(* Logix 5000 AddOnInstructionDefinition export Banner_S15C_B21_Param_v4; software revision 33.00 *)

TYPE Banner_Black_Host_Out_Mirroring :
STRUCT
   Enable : SINT;   // 0=Disabled, 1=Enabled
   Port_Selection : SINT;   // 0=Port 1
   Channel_Selection : SINT;   // 0=Discrete 1, 1=Discrete 2
   Inversion : SINT;   // 0=Not Inverted, 1=Inverted
   Polarity : SINT;   // 0=NPN Output, 1=PNP Output
   Output_Type : SINT;   // 1=Output Open Collector, 2=Output Push Pull
END_STRUCT
END_TYPE

TYPE Banner_Direct_v4 :
STRUCT
   Master_Cycle_Time : INT;
   Min_Cycle_Time : INT;
   M_Sequence_Capability : INT;
   IO_Link_Version_ID : INT;
   Process_Data_Input_Length : INT;
   Process_Data_Output_Length : INT;
   Combined_Vendor_ID : DINT;   // IO-Link Vendor ID
   Vendor_ID1 : INT;
   Vendor_ID2 : INT;
   Combined_Device_ID : DINT;   // IO-Link Device ID
   Device_ID1 : INT;
   Device_ID2 : INT;
   Device_ID3 : INT;
END_STRUCT
END_TYPE

TYPE Banner_Discrete_Host_Out_Mirroring_Cfg :
STRUCT
   Enable : SINT;   // 0=Disabled, 1=Enabled.
   Port_Selection : SINT;   // 0=Port 1
   Channel_Selection : SINT;   // 0=Discrete 1, 1=Discrete 2.
   Mirroring_Inversion : SINT;   // 0=Not Inverted, 1=Inverted.
   Mirroring_Polarity : SINT;   // 0=NPN Output, 1=PNP Output.
   Output_Type : SINT;   // 0=Output with Internal Pull Up / Down, 1=Output Open Collector, 2=Output Push Pull.
END_STRUCT
END_TYPE

TYPE Banner_IO_Metrics_v4 :
STRUCT
   Port_1_DI1_Count : DINT;
   Port_1_DI1_Duration : DINT;
   Port_1_DI1_Events_per_Minute : DINT;
   Port_1_DI1_Counts_per_Minute : DINT;
   Port_1_DI1_Totalizer_Counter : DINT;
   Port_1_DI2_Count : DINT;
   Port_1_DI2_Duration : DINT;
   Port_1_DI2_Events_per_Minute : DINT;
   Port_1_DI2_Counts_per_Minute : DINT;
   Port_1_DI2_Totalizer_Counter : DINT;
END_STRUCT
END_TYPE

TYPE Banner_IOL_Port_v4 :   // UDT that has all of the data items necessary to communicate with a specific Port on a IO-Link Master
STRUCT
   Port_Controlled : INT;   // Each bit represents a port on an IO-Link Master. Set to 1 to tell AOI to control that port.
   Port_Activate : INT;   // Each bit represents a port on an IO-Link Master. When ON that port will process any commands in queue.
   Port_Read : INT;   // Each bit represents a port on an IO-Link Master. Used to determine when device AOI has requested a Read command.
   Port_Write : INT;   // Each bit represents a port on an IO-Link Master. Used to determine when device AOI has requested a Write command.
   Port_RW_Complete : INT;   // Each bit represents a port on an IO-Link Master. Tells device AOI that Read or Write request has been completed.
   Port_Device_Read : INT;
   Data_Transfer : SINT[190];   // Array to transfer data from IO-Master to device AOIs.
END_STRUCT
END_TYPE

TYPE Banner_S15C_B21_Port_Config_v4 :
STRUCT
   DI1_IO_Selection : SINT;   // 0=NPN, 1=PNP
   DI1_Delay_Mode : SINT;   // 0=Disabled, 1=On Off Delay, 2=On One-Shot, 3=Off One-Shot, 4=On Pulse Stretcher, 5=Off Pulse Stretcher, 6=Totalizer
   DI1_Delay_Timer_1 : DINT;   // On Delay, One-Shot, Pulse Stretcher or Totalizer count.
   DI1_Delay_Timer_2 : DINT;   // Off Delay or Totalizer count.
   DI2_IO_Selection : SINT;   // 0=NPN, 1=PNP
   DI2_Delay_Mode : SINT;   // 0=Disabled, 1=On Off Delay, 2=On One-Shot, 3=Off One-Shot, 4=On Pulse Stretcher, 5=Off Pulse Stretcher, 6=Totalizer
   DI2_Delay_Timer_1 : DINT;   // On Delay, One-Shot, Pulse Stretcher or Totalizer count.
   DI2_Delay_Timer_2 : DINT;   // Off Delay or Totalizer count.
   Mirroring_Enable : SINT;   // 0=Disabled, 1=Enabled
   Mirroring_Port_Selection : SINT;   // 0 = Port 1
   Mirroring_Channel_Selection : SINT;   // 0=Discrete 1, 1=Discrete 2.
   Mirroring_Inversion : SINT;   // 0=Not Inverted, 1=Inverted
   Counts_per_Minute_Mode : SINT;   // 0=Slow, 1=Medium, 2=Fast
END_STRUCT
END_TYPE

TYPE Banner_S15C_B21_RD_v4 :   // All of the read parameters for a S15C unit.
STRUCT
   Direct : Banner_Direct_v4;
   Serial_Number : STRING;
   Product_Name : STRING;
   All_Time_Run_Time : DINT;   // Current All Time Run Timer.
   IO_Metrics : Banner_IO_Metrics_v4;
END_STRUCT
END_TYPE

TYPE Banner_S15C_B21_v4 :   // All of the parameters for a S15C.
STRUCT
   Initial_Global_Read : BOOL;   // Determines if all of the IO-Link data has been read into the PLC yet
   Command : INT;   // Value placed in here will activate a read or write to a specifc IO-Link Index
   Read : Banner_S15C_B21_RD_v4;   // Read Only Data
   Write : Banner_S15C_B21_WD_v4;   // Write Data
   Archive : Banner_S15C_B21_WD_v4;   // Archive Data
   Reset : BOOL;   // Resets AOI. This will force a complete parameter read of the sensor.
END_STRUCT
END_TYPE

TYPE Banner_S15C_B21_VSC_v4 :   // Vendor Specific Configuration Parameter Data for S15C-B21 unit.
STRUCT
   PDI1_Metric_Selection : SINT;   // 0 = Disabled, 1 = Count, 2 = Duration, 3 = Events per Minute
   PDI1_Port_Selection : SINT;   // 0 = Port 1
   PDI1_Channel_Selection : SINT;   // 0 = Discrete 1, 1 = Discrete 2
   PDI2_Metric_Selection : SINT;   // 0 = Disabled, 1 = Count, 2 = Duration, 3 = Events per Minute
   PDI2_Port_Selection : SINT;   // 0 = Port 1
   PDI2_Channel_Selection : SINT;   // 0 = Discrete 1, 1 = Discrete 2
   PDI3_Metric_Selection : SINT;   // 0 = Disabled, 1 = Count, 2 = Duration, 3 = Events per Minute
   PDI3_Port_Selection : SINT;   // 0 = Port 1
   PDI3_Channel_Selection : SINT;   // 0 = Discrete 1, 1 = Discrete 2
   PDI4_Metric_Selection : SINT;   // 0 = Disabled, 1 = Count, 2 = Duration, 3 = Events per Minute
   PDI4_Port_Selection : SINT;   // 0 = Port 1
   PDI4_Channel_Selection : SINT;   // 0 = Discrete 1, 1 = Discrete 2
END_STRUCT
END_TYPE

TYPE Banner_S15C_B21_WD_v4 :   // UDT that stores the Write Data for a S15C unit.
STRUCT
   System_Command : INT;   // See IODD file for list of commands that can be activated via the System Command interface
   Parameter_Access_Lock : SINT;   // Write access to all parameters is prohibited while value is 1. Only this parameter can be adjusted when value is 1.
   Data_Storage_Lock : SINT;   // Automatic data storage is disabled when this value is equal to 1. Read access is not affected.
   Local_Parameterization_Lock : SINT;   // Parameterization via local control elements on device is disabled.
   Local_User_Interface_Lock : SINT;   // Operation of local user interface is disabled.
   Resetable_Run_Time : DINT;   // Current Resetable Run Timer.
   VSC : Banner_S15C_B21_VSC_v4;
   All_Time_Run_Time_Event_Time : DINT;   // Time before an Event is generated. 0 = disable all-time event.
   Resetable_Run_Time_Event_Time : DINT;   // Time before an Event is generated. 0 = disable run time event.
   Port_1_Discrete_1 : SINT;   // 1 = Reset Activate
   Port_1_Discrete_2 : SINT;   // 1 = Reset Activate
   Port_1_Discrete_1_Reset_Count : DINT;
   Port_1_Discrete_2_Reset_Count : DINT;
   Port_1_Configuration : Banner_S15C_B21_Port_Config_v4;
   Mirroring_Config : Banner_Discrete_Host_Out_Mirroring_Cfg;
   Black_Mirroring_Config : Banner_Black_Host_Out_Mirroring;
END_STRUCT
END_TYPE

ADD_ON_INSTRUCTION Banner_S15C_B21_Param_v4   (* revision 4.3, vendor Banner Engineering *)
// AOI to read and write parameter data to an IO-Link S15C-B21.
VAR_IN_OUT
   S15C : Banner_S15C_B21_v4; {required}
   Port_Data : Banner_IOL_Port_v4; {required}
END_VAR
VAR_INPUT
   Port : DINT; {required}
END_VAR
VAR
   Local_Control : DINT; {access None}
   Global_Read_Command_Value : INT; {access None}
   Global_Write_Command_Value : INT; {access None}
   Error_Generated : BOOL; {access None}
   Command_Being_Processed : BOOL; {access None}
   Index_Write_Inprocess : INT; {access None}
   Index_Write_Control : INT; {access None}
   Update_Archive : BOOL; {access None}
   Inprocess_Index : DINT; {access None}
END_VAR

ROUTINE Logic   (* ladder *)
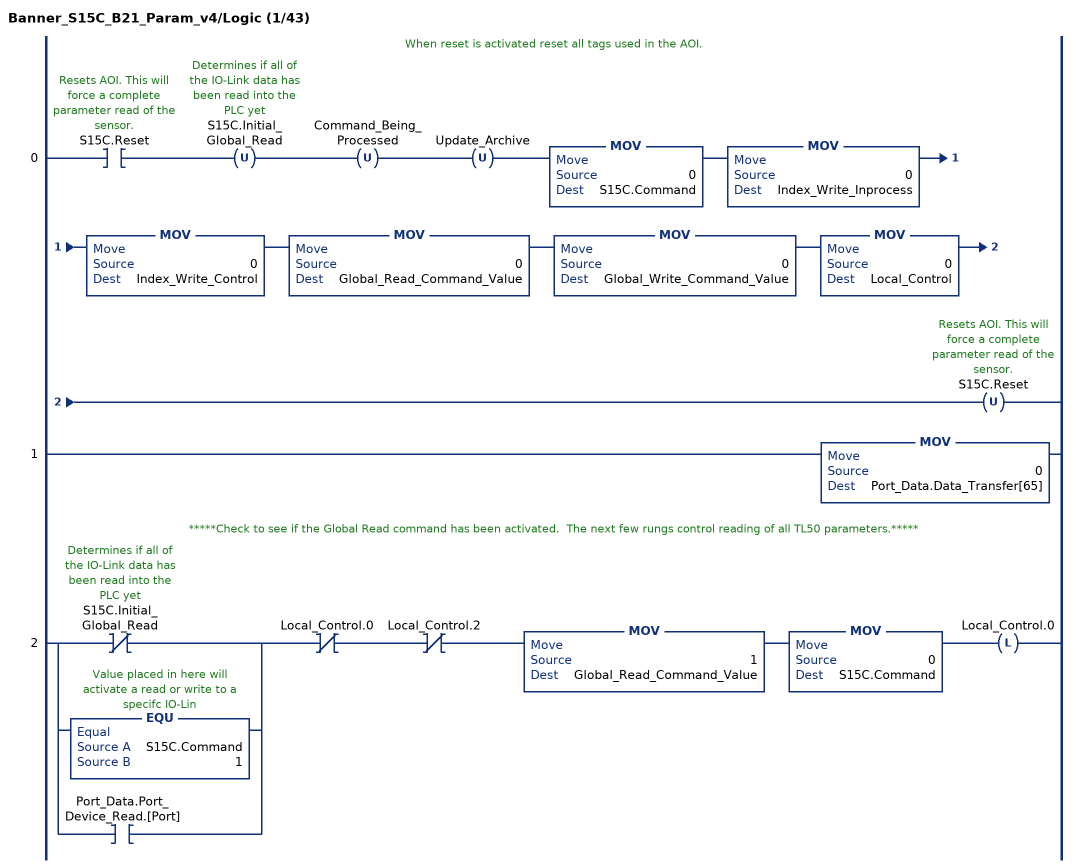
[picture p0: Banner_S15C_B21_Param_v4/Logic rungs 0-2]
   // When reset is activated reset all tags used in the AOI.
   0: XIC(S15C.Reset)OTU(S15C.Initial_Global_Read)OTU(Command_Being_Processed)OTU(Update_Archive)MOV(0,S15C.Command)MOV(0,Index_Write_Inprocess)MOV(0,Index_Write_Control)MOV(0,Global_Read_Command_Value)MOV(0,Global_Write_Command_Value)MOV(0,Local_Control)OTU(S15C.Reset);
   1: MOV(0,Port_Data.Data_Transfer[65]);
   // *****Check to see if the Global Read command has been activated.  The next few rungs control reading of all TL50 parameters.*****
   2: [XIO(S15C.Initial_Global_Read) ,EQU(S15C.Command,1) ,XIC(Port_Data.Port_Device_Read.[Port]) ]XIO(Local_Control.0)XIO(Local_Control.2)MOV(1,Global_Read_Command_Value)MOV(0,S15C.Command)OTL(Local_Control.0);
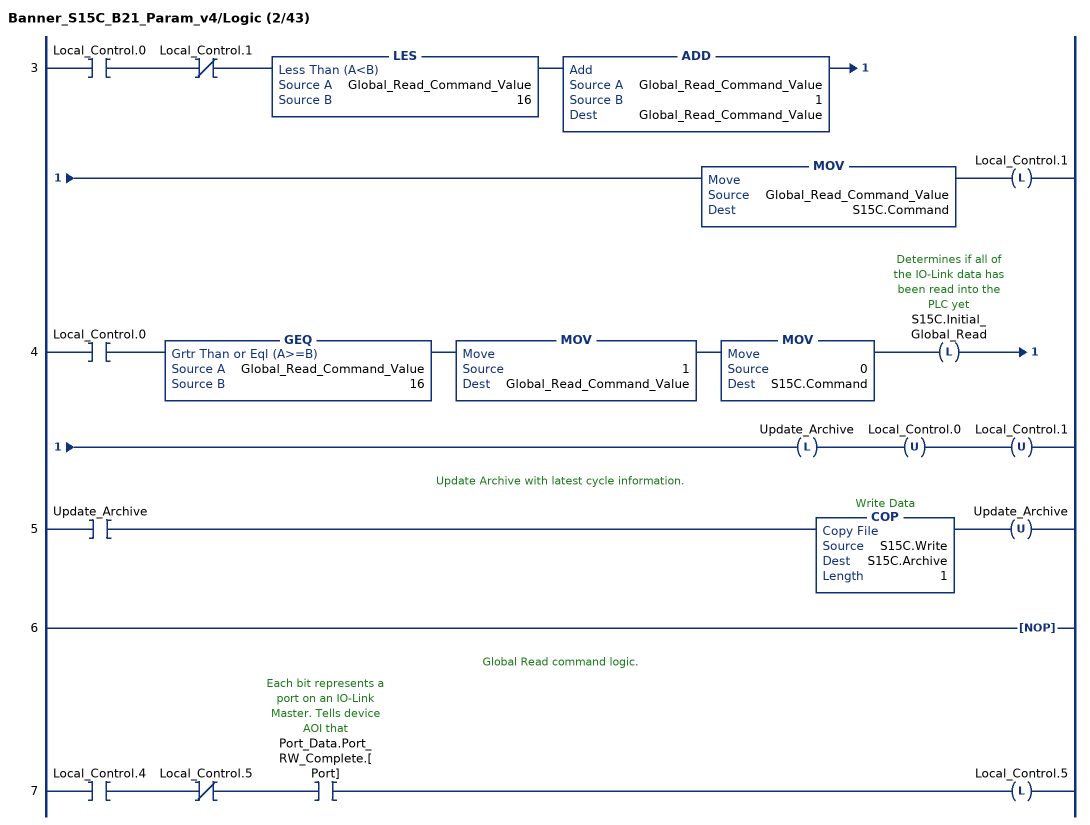
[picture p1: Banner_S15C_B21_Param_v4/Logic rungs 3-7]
   3: XIC(Local_Control.0)XIO(Local_Control.1)LES(Global_Read_Command_Value,16)ADD(Global_Read_Command_Value,1,Global_Read_Command_Value)MOV(Global_Read_Command_Value,S15C.Command)OTL(Local_Control.1);
   4: XIC(Local_Control.0)GEQ(Global_Read_Command_Value,16)MOV(1,Global_Read_Command_Value)MOV(0,S15C.Command)OTL(S15C.Initial_Global_Read)OTL(Update_Archive)OTU(Local_Control.0)OTU(Local_Control.1);
   // Update Archive with latest cycle information.
   5: XIC(Update_Archive)COP(S15C.Write,S15C.Archive,1)OTU(Update_Archive);
   6: NOP();
   // Global Read command logic.
   7: XIC(Local_Control.4)XIO(Local_Control.5)XIC(Port_Data.Port_RW_Complete.[Port])OTL(Local_Control.5);
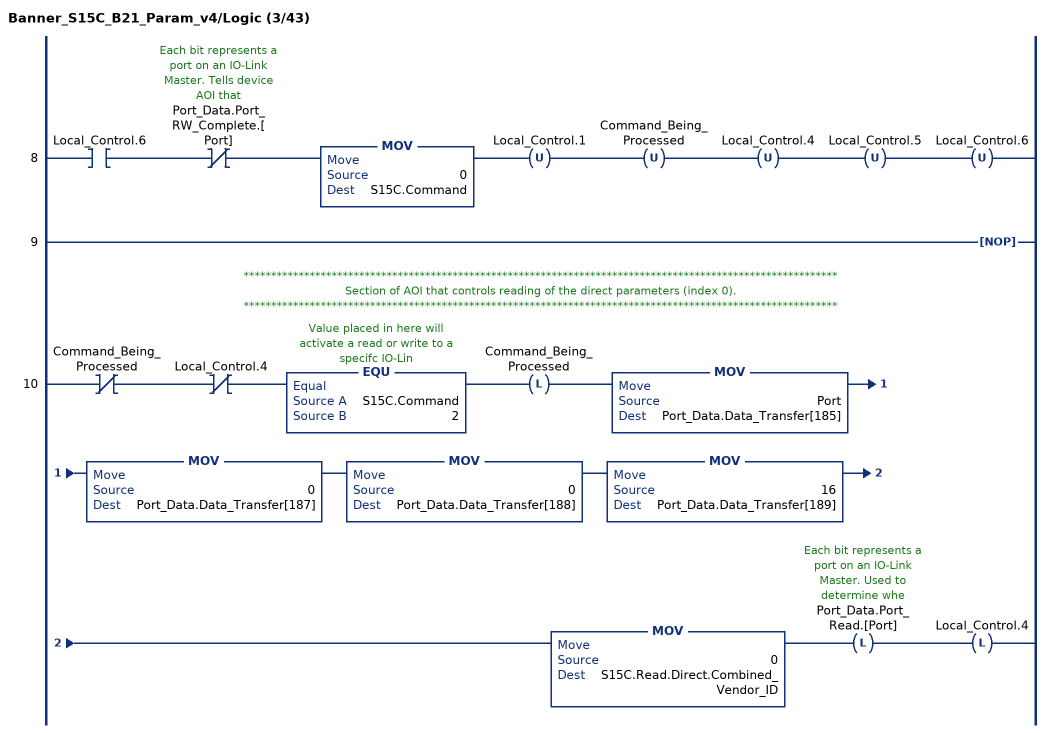
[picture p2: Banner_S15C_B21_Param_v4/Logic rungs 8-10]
   8: XIC(Local_Control.6)XIO(Port_Data.Port_RW_Complete.[Port])MOV(0,S15C.Command)OTU(Local_Control.1)OTU(Command_Being_Processed)OTU(Local_Control.4)OTU(Local_Control.5)OTU(Local_Control.6);
   9: NOP();
   // ************************************************************************************************************
   // Section of AOI that controls reading of the direct parameters (index 0).
   // ************************************************************************************************************
   10: XIO(Command_Being_Processed)XIO(Local_Control.4)EQU(S15C.Command,2)OTL(Command_Being_Processed)MOV(Port,Port_Data.Data_Transfer[185])MOV(0,Port_Data.Data_Transfer[187])MOV(0,Port_Data.Data_Transfer[188])MOV(16,Port_Data.Data_Transfer[189])MOV(0,S15C.Read.Direct.Combined_Vendor_ID)OTL(Port_Data.Port_Read.[Port])OTL(Local_Control.4);
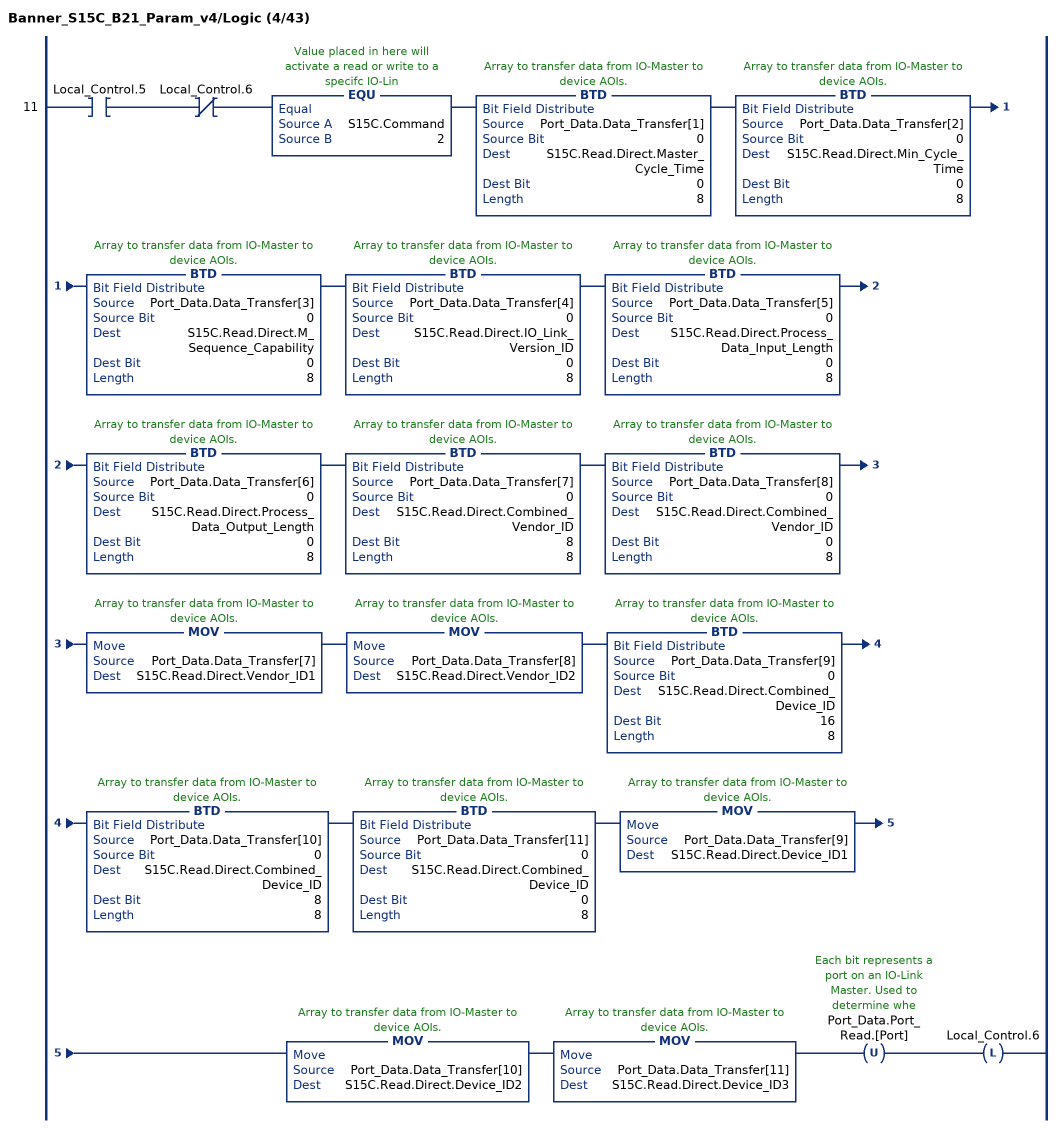
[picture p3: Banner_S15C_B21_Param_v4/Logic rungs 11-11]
   11: XIC(Local_Control.5)XIO(Local_Control.6)EQU(S15C.Command,2)BTD(Port_Data.Data_Transfer[1],0,S15C.Read.Direct.Master_Cycle_Time,0,8)BTD(Port_Data.Data_Transfer[2],0,S15C.Read.Direct.Min_Cycle_Time,0,8)BTD(Port_Data.Data_Transfer[3],0,S15C.Read.Direct.M_Sequence_Capability,0,8)BTD(Port_Data.Data_Transfer[4],0,S15C.Read.Direct.IO_Link_Version_ID,0,8)BTD(Port_Data.Data_Transfer[5],0,S15C.Read.Direct.Process_Data_Input_Length,0,8)BTD(Port_Data.Data_Transfer[6],0,S15C.Read.Direct.Process_Data_Output_Length,0,8)BTD(Port_Data.Data_Transfer[7],0,S15C.Read.Direct.Combined_Vendor_ID,8,8)BTD(Port_Data.Data_Transfer[8],0,S15C.Read.Direct.Combined_Vendor_ID,0,8)MOV(Port_Data.Data_Transfer[7],S15C.Read.Direct.Vendor_ID1)MOV(Port_Data.Data_Transfer[8],S15C.Read.Direct.Vendor_ID2)BTD(Port_Data.Data_Transfer[9],0,S15C.Read.Direct.Combined_Device_ID,16,8)BTD(Port_Data.Data_Transfer[10],0,S15C.Read.Direct.Combined_Device_ID,8,8)BTD(Port_Data.Data_Transfer[11],0,S15C.Read.Direct.Combined_Device_ID,0,8)MOV(Port_Data.Data_Transfer[9],S15C.Read.Direct.Device_ID1)MOV(Port_Data.Data_Transfer[10],S15C.Read.Direct.Device_ID2)MOV(Port_Data.Data_Transfer[11],S15C.Read.Direct.Device_ID3)OTU(Port_Data.Port_Read.[Port])OTL(Local_Control.6);
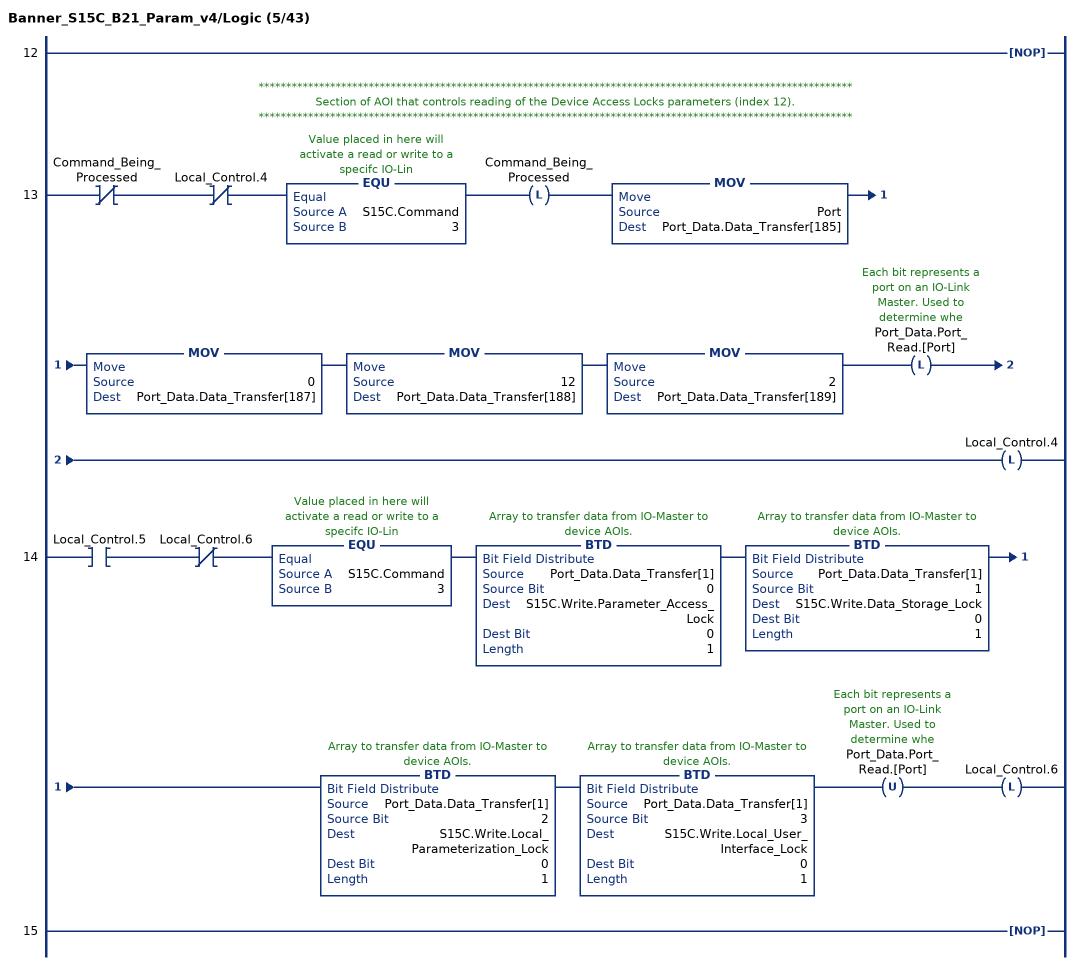
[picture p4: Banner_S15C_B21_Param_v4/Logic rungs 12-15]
   12: NOP();
   // ************************************************************************************************************
   // Section of AOI that controls reading of the Device Access Locks parameters (index 12).
   // ************************************************************************************************************
   13: XIO(Command_Being_Processed)XIO(Local_Control.4)EQU(S15C.Command,3)OTL(Command_Being_Processed)MOV(Port,Port_Data.Data_Transfer[185])MOV(0,Port_Data.Data_Transfer[187])MOV(12,Port_Data.Data_Transfer[188])MOV(2,Port_Data.Data_Transfer[189])OTL(Port_Data.Port_Read.[Port])OTL(Local_Control.4);
   14: XIC(Local_Control.5)XIO(Local_Control.6)EQU(S15C.Command,3)BTD(Port_Data.Data_Transfer[1],0,S15C.Write.Parameter_Access_Lock,0,1)BTD(Port_Data.Data_Transfer[1],1,S15C.Write.Data_Storage_Lock,0,1)BTD(Port_Data.Data_Transfer[1],2,S15C.Write.Local_Parameterization_Lock,0,1)BTD(Port_Data.Data_Transfer[1],3,S15C.Write.Local_User_Interface_Lock,0,1)OTU(Port_Data.Port_Read.[Port])OTL(Local_Control.6);
   15: NOP();
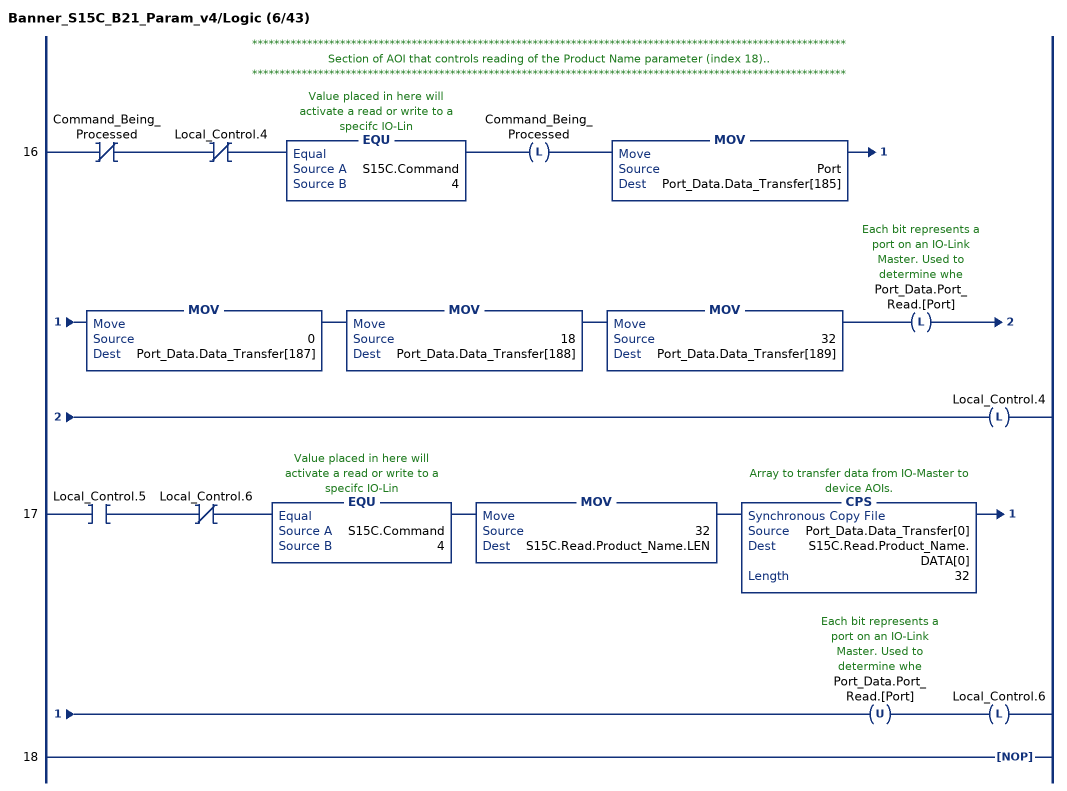
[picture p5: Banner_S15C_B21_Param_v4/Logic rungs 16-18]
   // ************************************************************************************************************
   // Section of AOI that controls reading of the Product Name parameter (index 18)..
   // ************************************************************************************************************
   16: XIO(Command_Being_Processed)XIO(Local_Control.4)EQU(S15C.Command,4)OTL(Command_Being_Processed)MOV(Port,Port_Data.Data_Transfer[185])MOV(0,Port_Data.Data_Transfer[187])MOV(18,Port_Data.Data_Transfer[188])MOV(32,Port_Data.Data_Transfer[189])OTL(Port_Data.Port_Read.[Port])OTL(Local_Control.4);
   17: XIC(Local_Control.5)XIO(Local_Control.6)EQU(S15C.Command,4)MOV(32,S15C.Read.Product_Name.LEN)CPS(Port_Data.Data_Transfer[0],S15C.Read.Product_Name.DATA[0],32)OTU(Port_Data.Port_Read.[Port])OTL(Local_Control.6);
   18: NOP();
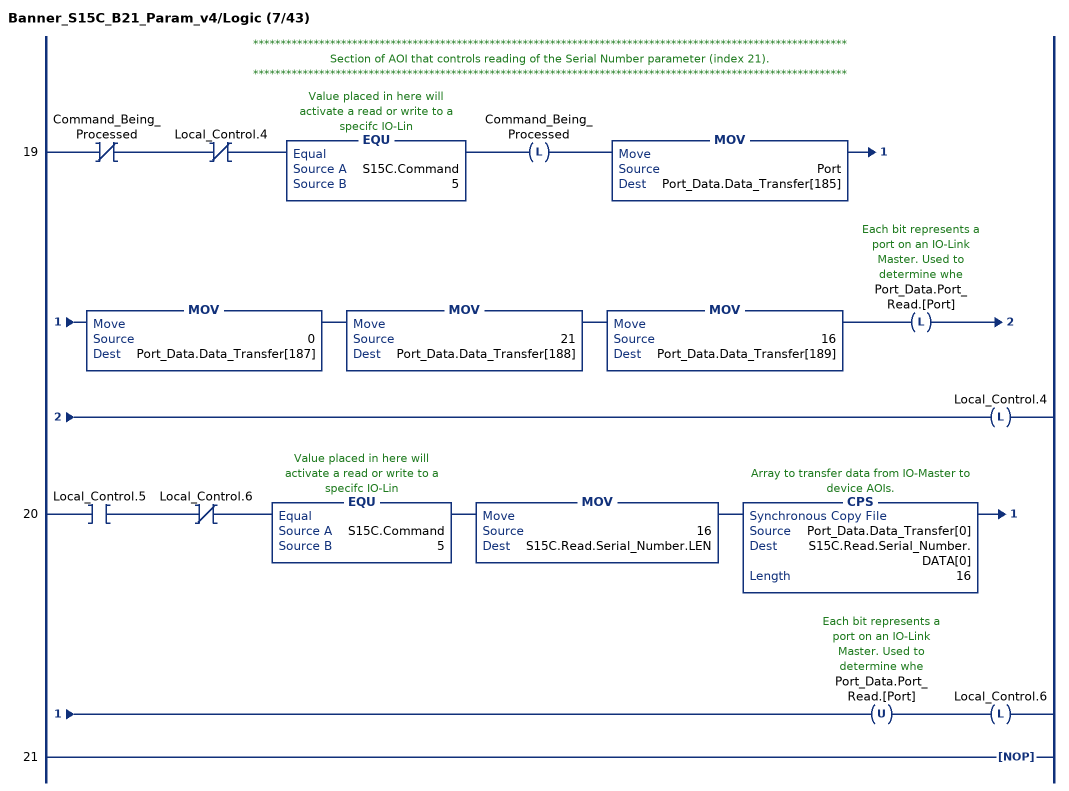
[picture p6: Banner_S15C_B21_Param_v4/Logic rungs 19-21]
   // ************************************************************************************************************
   // Section of AOI that controls reading of the Serial Number parameter (index 21).
   // ************************************************************************************************************
   19: XIO(Command_Being_Processed)XIO(Local_Control.4)EQU(S15C.Command,5)OTL(Command_Being_Processed)MOV(Port,Port_Data.Data_Transfer[185])MOV(0,Port_Data.Data_Transfer[187])MOV(21,Port_Data.Data_Transfer[188])MOV(16,Port_Data.Data_Transfer[189])OTL(Port_Data.Port_Read.[Port])OTL(Local_Control.4);
   20: XIC(Local_Control.5)XIO(Local_Control.6)EQU(S15C.Command,5)MOV(16,S15C.Read.Serial_Number.LEN)CPS(Port_Data.Data_Transfer[0],S15C.Read.Serial_Number.DATA[0],16)OTU(Port_Data.Port_Read.[Port])OTL(Local_Control.6);
   21: NOP();
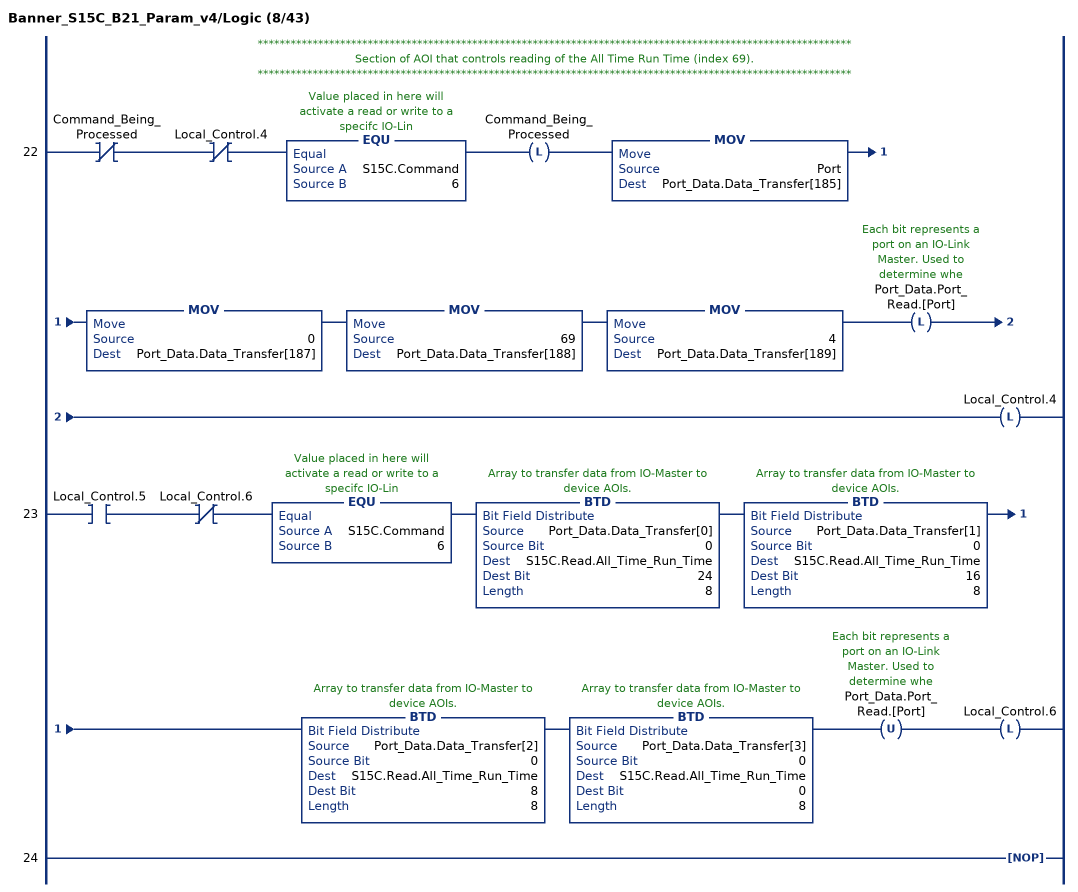
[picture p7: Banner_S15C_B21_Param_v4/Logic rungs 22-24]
   // ************************************************************************************************************
   // Section of AOI that controls reading of the All Time Run Time (index 69).
   // ************************************************************************************************************
   22: XIO(Command_Being_Processed)XIO(Local_Control.4)EQU(S15C.Command,6)OTL(Command_Being_Processed)MOV(Port,Port_Data.Data_Transfer[185])MOV(0,Port_Data.Data_Transfer[187])MOV(69,Port_Data.Data_Transfer[188])MOV(4,Port_Data.Data_Transfer[189])OTL(Port_Data.Port_Read.[Port])OTL(Local_Control.4);
   23: XIC(Local_Control.5)XIO(Local_Control.6)EQU(S15C.Command,6)BTD(Port_Data.Data_Transfer[0],0,S15C.Read.All_Time_Run_Time,24,8)BTD(Port_Data.Data_Transfer[1],0,S15C.Read.All_Time_Run_Time,16,8)BTD(Port_Data.Data_Transfer[2],0,S15C.Read.All_Time_Run_Time,8,8)BTD(Port_Data.Data_Transfer[3],0,S15C.Read.All_Time_Run_Time,0,8)OTU(Port_Data.Port_Read.[Port])OTL(Local_Control.6);
   24: NOP();
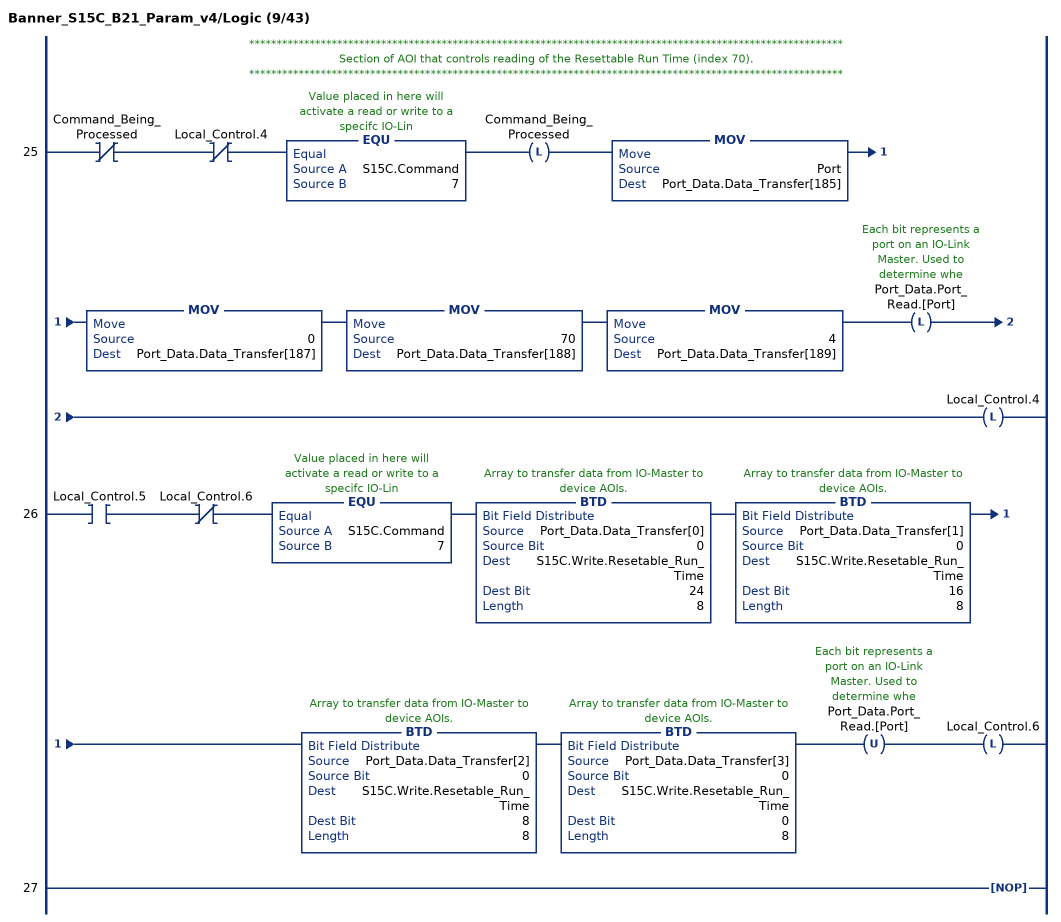
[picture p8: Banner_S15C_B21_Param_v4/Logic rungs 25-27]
   // ************************************************************************************************************
   // Section of AOI that controls reading of the Resettable Run Time (index 70).
   // ************************************************************************************************************
   25: XIO(Command_Being_Processed)XIO(Local_Control.4)EQU(S15C.Command,7)OTL(Command_Being_Processed)MOV(Port,Port_Data.Data_Transfer[185])MOV(0,Port_Data.Data_Transfer[187])MOV(70,Port_Data.Data_Transfer[188])MOV(4,Port_Data.Data_Transfer[189])OTL(Port_Data.Port_Read.[Port])OTL(Local_Control.4);
   26: XIC(Local_Control.5)XIO(Local_Control.6)EQU(S15C.Command,7)BTD(Port_Data.Data_Transfer[0],0,S15C.Write.Resetable_Run_Time,24,8)BTD(Port_Data.Data_Transfer[1],0,S15C.Write.Resetable_Run_Time,16,8)BTD(Port_Data.Data_Transfer[2],0,S15C.Write.Resetable_Run_Time,8,8)BTD(Port_Data.Data_Transfer[3],0,S15C.Write.Resetable_Run_Time,0,8)OTU(Port_Data.Port_Read.[Port])OTL(Local_Control.6);
   27: NOP();
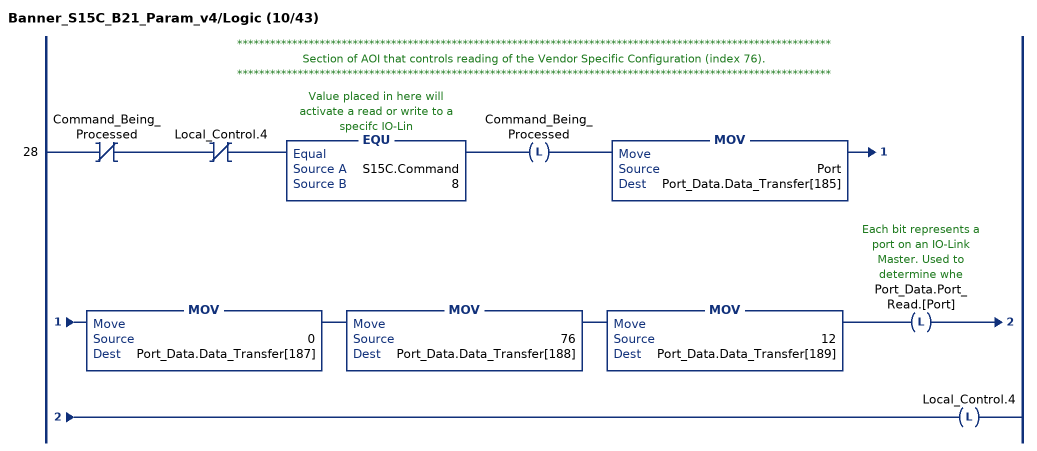
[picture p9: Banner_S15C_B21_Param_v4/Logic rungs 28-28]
   // ************************************************************************************************************
   // Section of AOI that controls reading of the Vendor Specific Configuration (index 76).
   // ************************************************************************************************************
   28: XIO(Command_Being_Processed)XIO(Local_Control.4)EQU(S15C.Command,8)OTL(Command_Being_Processed)MOV(Port,Port_Data.Data_Transfer[185])MOV(0,Port_Data.Data_Transfer[187])MOV(76,Port_Data.Data_Transfer[188])MOV(12,Port_Data.Data_Transfer[189])OTL(Port_Data.Port_Read.[Port])OTL(Local_Control.4);
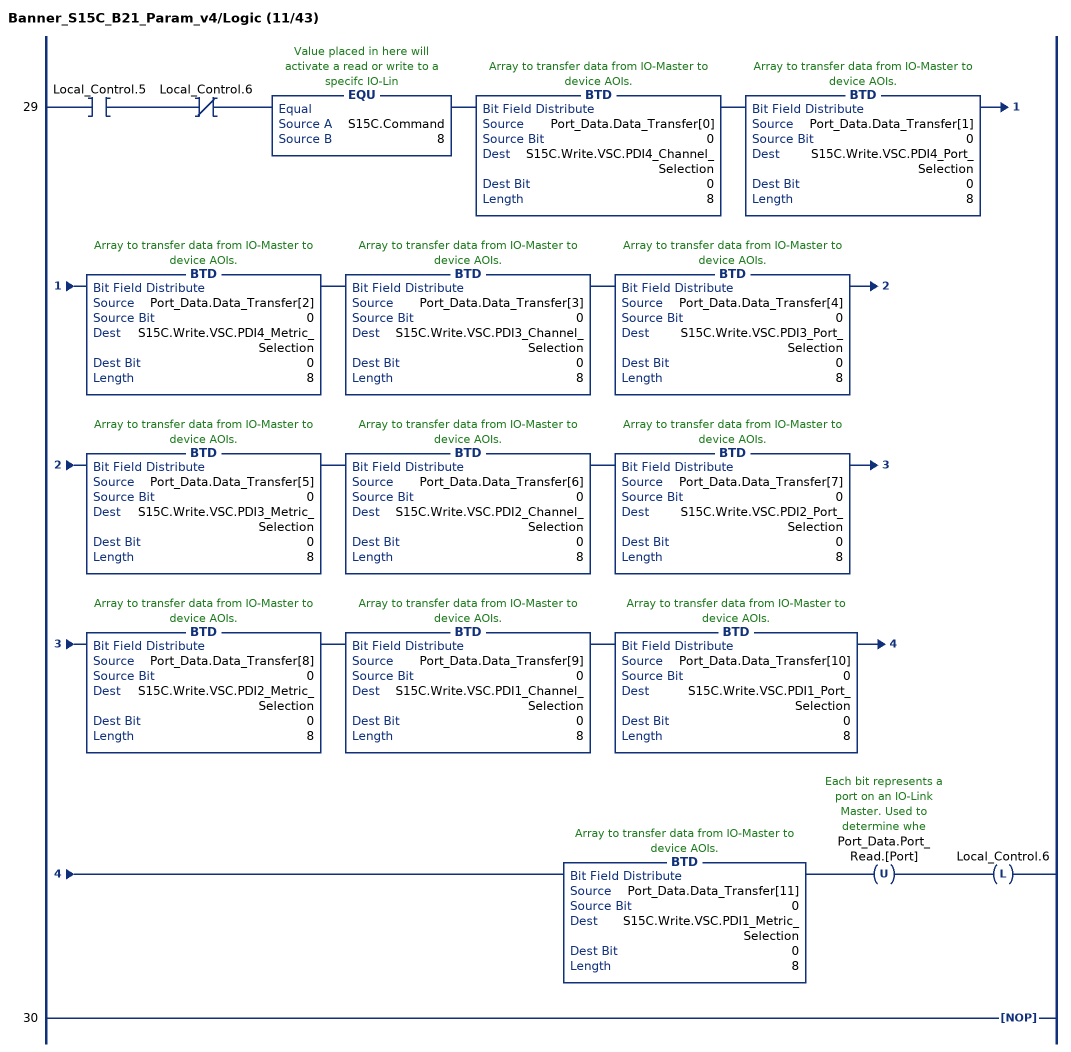
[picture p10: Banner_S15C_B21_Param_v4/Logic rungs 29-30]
   29: XIC(Local_Control.5)XIO(Local_Control.6)EQU(S15C.Command,8)BTD(Port_Data.Data_Transfer[0],0,S15C.Write.VSC.PDI4_Channel_Selection,0,8)BTD(Port_Data.Data_Transfer[1],0,S15C.Write.VSC.PDI4_Port_Selection,0,8)BTD(Port_Data.Data_Transfer[2],0,S15C.Write.VSC.PDI4_Metric_Selection,0,8)BTD(Port_Data.Data_Transfer[3],0,S15C.Write.VSC.PDI3_Channel_Selection,0,8)BTD(Port_Data.Data_Transfer[4],0,S15C.Write.VSC.PDI3_Port_Selection,0,8)BTD(Port_Data.Data_Transfer[5],0,S15C.Write.VSC.PDI3_Metric_Selection,0,8)BTD(Port_Data.Data_Transfer[6],0,S15C.Write.VSC.PDI2_Channel_Selection,0,8)BTD(Port_Data.Data_Transfer[7],0,S15C.Write.VSC.PDI2_Port_Selection,0,8)BTD(Port_Data.Data_Transfer[8],0,S15C.Write.VSC.PDI2_Metric_Selection,0,8)BTD(Port_Data.Data_Transfer[9],0,S15C.Write.VSC.PDI1_Channel_Selection,0,8)BTD(Port_Data.Data_Transfer[10],0,S15C.Write.VSC.PDI1_Port_Selection,0,8)BTD(Port_Data.Data_Transfer[11],0,S15C.Write.VSC.PDI1_Metric_Selection,0,8)OTU(Port_Data.Port_Read.[Port])OTL(Local_Control.6);
   30: NOP();
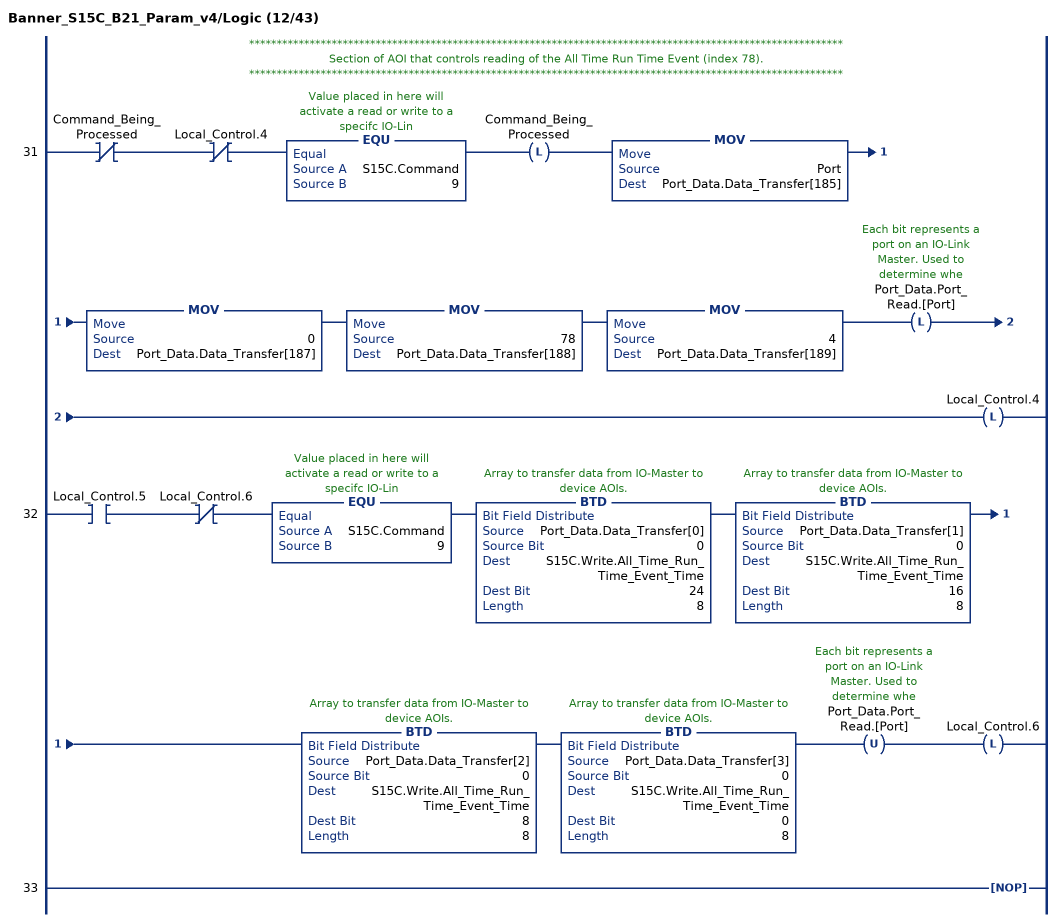
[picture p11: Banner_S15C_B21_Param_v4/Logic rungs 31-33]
   // ************************************************************************************************************
   // Section of AOI that controls reading of the All Time Run Time Event (index 78).
   // ************************************************************************************************************
   31: XIO(Command_Being_Processed)XIO(Local_Control.4)EQU(S15C.Command,9)OTL(Command_Being_Processed)MOV(Port,Port_Data.Data_Transfer[185])MOV(0,Port_Data.Data_Transfer[187])MOV(78,Port_Data.Data_Transfer[188])MOV(4,Port_Data.Data_Transfer[189])OTL(Port_Data.Port_Read.[Port])OTL(Local_Control.4);
   32: XIC(Local_Control.5)XIO(Local_Control.6)EQU(S15C.Command,9)BTD(Port_Data.Data_Transfer[0],0,S15C.Write.All_Time_Run_Time_Event_Time,24,8)BTD(Port_Data.Data_Transfer[1],0,S15C.Write.All_Time_Run_Time_Event_Time,16,8)BTD(Port_Data.Data_Transfer[2],0,S15C.Write.All_Time_Run_Time_Event_Time,8,8)BTD(Port_Data.Data_Transfer[3],0,S15C.Write.All_Time_Run_Time_Event_Time,0,8)OTU(Port_Data.Port_Read.[Port])OTL(Local_Control.6);
   33: NOP();
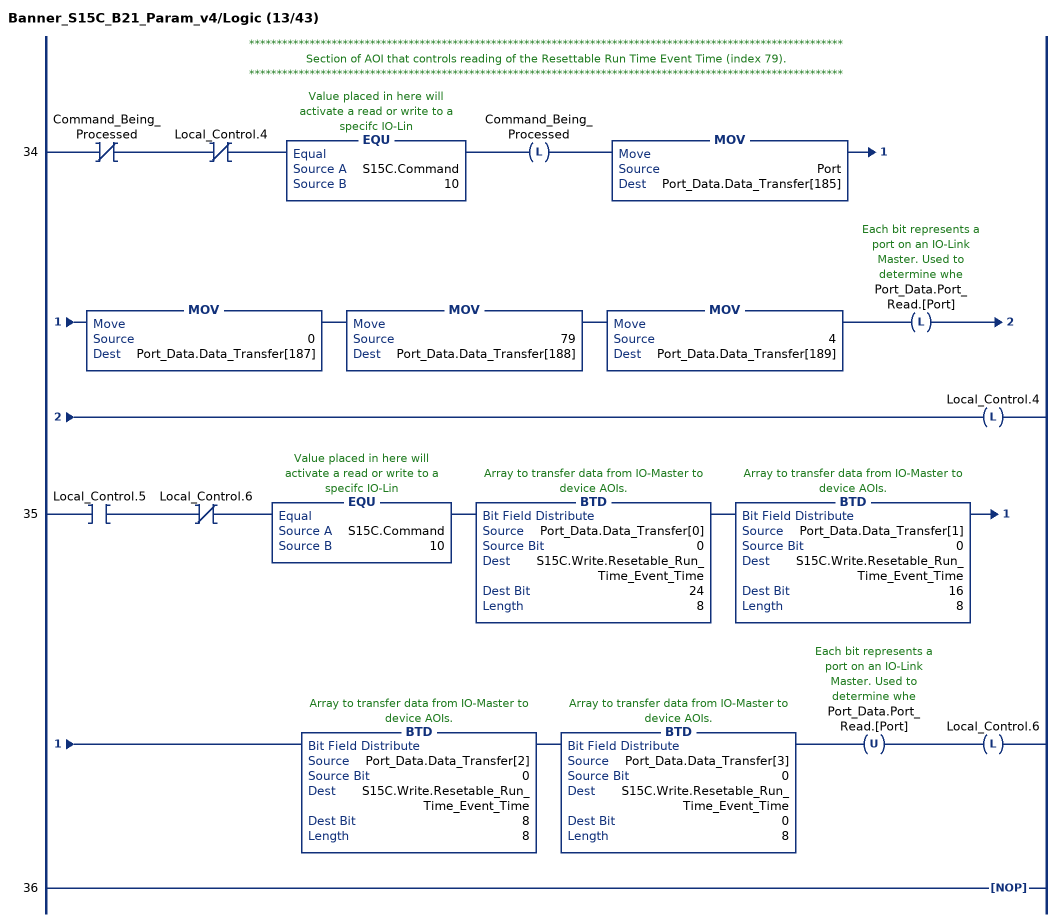
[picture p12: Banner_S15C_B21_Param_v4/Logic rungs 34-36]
   // ************************************************************************************************************
   // Section of AOI that controls reading of the Resettable Run Time Event Time (index 79).
   // ************************************************************************************************************
   34: XIO(Command_Being_Processed)XIO(Local_Control.4)EQU(S15C.Command,10)OTL(Command_Being_Processed)MOV(Port,Port_Data.Data_Transfer[185])MOV(0,Port_Data.Data_Transfer[187])MOV(79,Port_Data.Data_Transfer[188])MOV(4,Port_Data.Data_Transfer[189])OTL(Port_Data.Port_Read.[Port])OTL(Local_Control.4);
   35: XIC(Local_Control.5)XIO(Local_Control.6)EQU(S15C.Command,10)BTD(Port_Data.Data_Transfer[0],0,S15C.Write.Resetable_Run_Time_Event_Time,24,8)BTD(Port_Data.Data_Transfer[1],0,S15C.Write.Resetable_Run_Time_Event_Time,16,8)BTD(Port_Data.Data_Transfer[2],0,S15C.Write.Resetable_Run_Time_Event_Time,8,8)BTD(Port_Data.Data_Transfer[3],0,S15C.Write.Resetable_Run_Time_Event_Time,0,8)OTU(Port_Data.Port_Read.[Port])OTL(Local_Control.6);
   36: NOP();
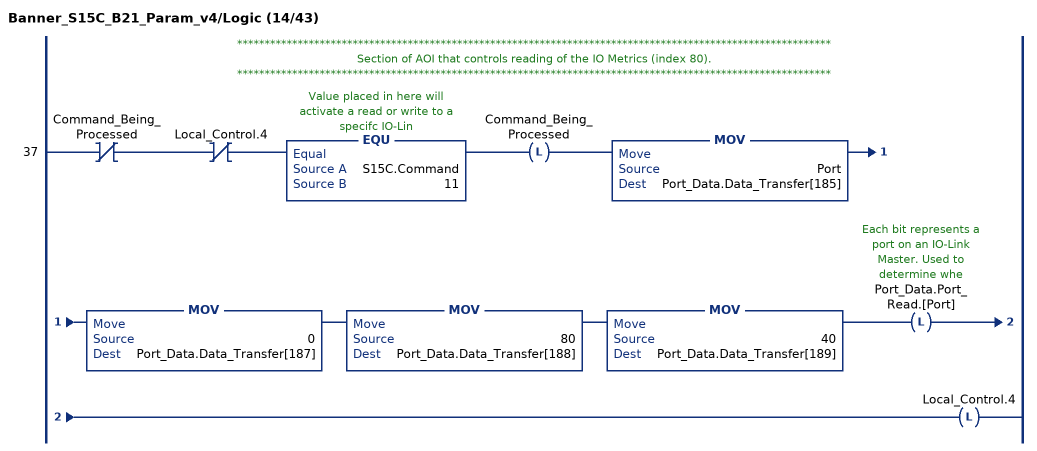
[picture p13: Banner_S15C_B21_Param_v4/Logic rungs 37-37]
   // ************************************************************************************************************
   // Section of AOI that controls reading of the IO Metrics (index 80).
   // ************************************************************************************************************
   37: XIO(Command_Being_Processed)XIO(Local_Control.4)EQU(S15C.Command,11)OTL(Command_Being_Processed)MOV(Port,Port_Data.Data_Transfer[185])MOV(0,Port_Data.Data_Transfer[187])MOV(80,Port_Data.Data_Transfer[188])MOV(40,Port_Data.Data_Transfer[189])OTL(Port_Data.Port_Read.[Port])OTL(Local_Control.4);
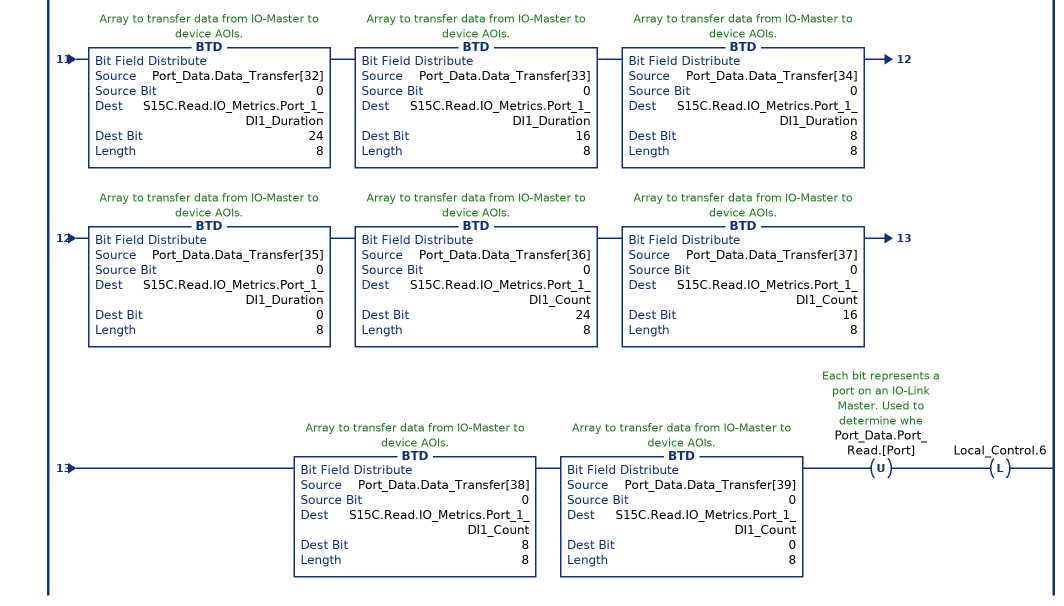
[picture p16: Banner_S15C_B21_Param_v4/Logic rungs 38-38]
   38: XIC(Local_Control.5)XIO(Local_Control.6)EQU(S15C.Command,11)BTD(Port_Data.Data_Transfer[0],0,S15C.Read.IO_Metrics.Port_1_DI2_Totalizer_Counter,24,8)BTD(Port_Data.Data_Transfer[1],0,S15C.Read.IO_Metrics.Port_1_DI2_Totalizer_Counter,16,8)BTD(Port_Data.Data_Transfer[2],0,S15C.Read.IO_Metrics.Port_1_DI2_Totalizer_Counter,8,8)BTD(Port_Data.Data_Transfer[3],0,S15C.Read.IO_Metrics.Port_1_DI2_Totalizer_Counter,0,8)BTD(Port_Data.Data_Transfer[4],0,S15C.Read.IO_Metrics.Port_1_DI2_Counts_per_Minute,24,8)BTD(Port_Data.Data_Transfer[5],0,S15C.Read.IO_Metrics.Port_1_DI2_Counts_per_Minute,16,8)BTD(Port_Data.Data_Transfer[6],0,S15C.Read.IO_Metrics.Port_1_DI2_Counts_per_Minute,8,8)BTD(Port_Data.Data_Transfer[7],0,S15C.Read.IO_Metrics.Port_1_DI2_Counts_per_Minute,0,8)BTD(Port_Data.Data_Transfer[8],0,S15C.Read.IO_Metrics.Port_1_DI2_Events_per_Minute,24,8)BTD(Port_Data.Data_Transfer[9],0,S15C.Read.IO_Metrics.Port_1_DI2_Events_per_Minute,16,8)BTD(Port_Data.Data_Transfer[10],0,S15C.Read.IO_Metrics.Port_1_DI2_Events_per_Minute,8,8)BTD(Port_Data.Data_Transfer[11],0,S15C.Read.IO_Metrics.Port_1_DI2_Events_per_Minute,0,8)BTD(Port_Data.Data_Transfer[12],0,S15C.Read.IO_Metrics.Port_1_DI2_Duration,24,8)BTD(Port_Data.Data_Transfer[13],0,S15C.Read.IO_Metrics.Port_1_DI2_Duration,16,8)BTD(Port_Data.Data_Transfer[14],0,S15C.Read.IO_Metrics.Port_1_DI2_Duration,8,8)BTD(Port_Data.Data_Transfer[15],0,S15C.Read.IO_Metrics.Port_1_DI2_Duration,0,8)BTD(Port_Data.Data_Transfer[16],0,S15C.Read.IO_Metrics.Port_1_DI2_Count,24,8)BTD(Port_Data.Data_Transfer[17],0,S15C.Read.IO_Metrics.Port_1_DI2_Count,16,8)BTD(Port_Data.Data_Transfer[18],0,S15C.Read.IO_Metrics.Port_1_DI2_Count,8,8)BTD(Port_Data.Data_Transfer[19],0,S15C.Read.IO_Metrics.Port_1_DI2_Count,0,8)BTD(Port_Data.Data_Transfer[20],0,S15C.Read.IO_Metrics.Port_1_DI1_Totalizer_Counter,24,8)BTD(Port_Data.Data_Transfer[21],0,S15C.Read.IO_Metrics.Port_1_DI1_Totalizer_Counter,16,8)BTD(Port_Data.Data_Transfer[22],0,S15C.Read.IO_Metrics.Port_1_DI1_Totalizer_Counter,8,8)BTD(Port_Data.Data_Transfer[23],0,S15C.Read.IO_Metrics.Port_1_DI1_Totalizer_Counter,0,8)BTD(Port_Data.Data_Transfer[24],0,S15C.Read.IO_Metrics.Port_1_DI1_Counts_per_Minute,24,8)BTD(Port_Data.Data_Transfer[25],0,S15C.Read.IO_Metrics.Port_1_DI1_Counts_per_Minute,16,8)BTD(Port_Data.Data_Transfer[26],0,S15C.Read.IO_Metrics.Port_1_DI1_Counts_per_Minute,8,8)BTD(Port_Data.Data_Transfer[27],0,S15C.Read.IO_Metrics.Port_1_DI1_Counts_per_Minute,0,8)BTD(Port_Data.Data_Transfer[28],0,S15C.Read.IO_Metrics.Port_1_DI1_Events_per_Minute,24,8)BTD(Port_Data.Data_Transfer[29],0,S15C.Read.IO_Metrics.Port_1_DI1_Events_per_Minute,16,8)BTD(Port_Data.Data_Transfer[30],0,S15C.Read.IO_Metrics.Port_1_DI1_Events_per_Minute,8,8)BTD(Port_Data.Data_Transfer[31],0,S15C.Read.IO_Metrics.Port_1_DI1_Events_per_Minute,0,8)BTD(Port_Data.Data_Transfer[32],0,S15C.Read.IO_Metrics.Port_1_DI1_Duration,24,8)BTD(Port_Data.Data_Transfer[33],0,S15C.Read.IO_Metrics.Port_1_DI1_Duration,16,8)BTD(Port_Data.Data_Transfer[34],0,S15C.Read.IO_Metrics.Port_1_DI1_Duration,8,8)BTD(Port_Data.Data_Transfer[35],0,S15C.Read.IO_Metrics.Port_1_DI1_Duration,0,8)BTD(Port_Data.Data_Transfer[36],0,S15C.Read.IO_Metrics.Port_1_DI1_Count,24,8)BTD(Port_Data.Data_Transfer[37],0,S15C.Read.IO_Metrics.Port_1_DI1_Count,16,8)BTD(Port_Data.Data_Transfer[38],0,S15C.Read.IO_Metrics.Port_1_DI1_Count,8,8)BTD(Port_Data.Data_Transfer[39],0,S15C.Read.IO_Metrics.Port_1_DI1_Count,0,8)OTU(Port_Data.Port_Read.[Port])OTL(Local_Control.6);
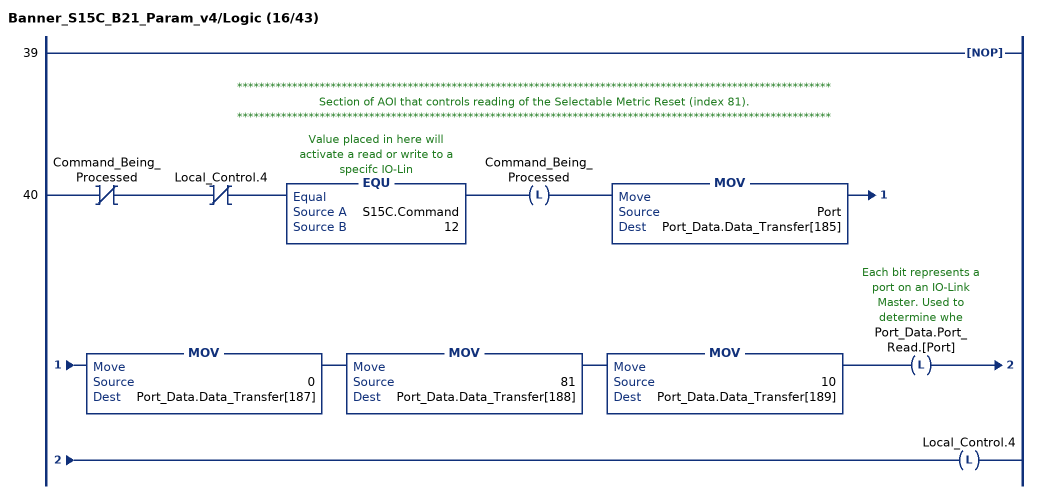
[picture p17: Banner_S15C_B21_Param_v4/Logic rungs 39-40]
   39: NOP();
   // ************************************************************************************************************
   // Section of AOI that controls reading of the Selectable Metric Reset (index 81).
   // ************************************************************************************************************
   40: XIO(Command_Being_Processed)XIO(Local_Control.4)EQU(S15C.Command,12)OTL(Command_Being_Processed)MOV(Port,Port_Data.Data_Transfer[185])MOV(0,Port_Data.Data_Transfer[187])MOV(81,Port_Data.Data_Transfer[188])MOV(10,Port_Data.Data_Transfer[189])OTL(Port_Data.Port_Read.[Port])OTL(Local_Control.4);
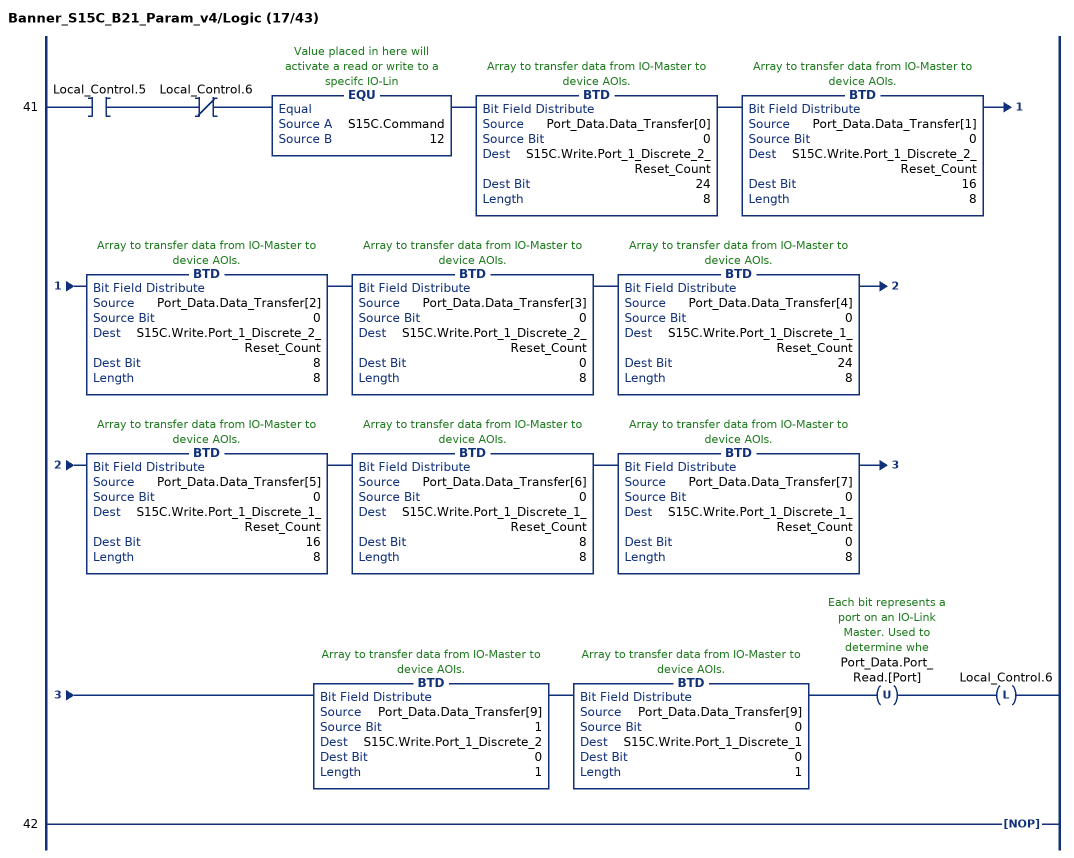
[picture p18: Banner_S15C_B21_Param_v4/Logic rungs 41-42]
   41: XIC(Local_Control.5)XIO(Local_Control.6)EQU(S15C.Command,12)BTD(Port_Data.Data_Transfer[0],0,S15C.Write.Port_1_Discrete_2_Reset_Count,24,8)BTD(Port_Data.Data_Transfer[1],0,S15C.Write.Port_1_Discrete_2_Reset_Count,16,8)BTD(Port_Data.Data_Transfer[2],0,S15C.Write.Port_1_Discrete_2_Reset_Count,8,8)BTD(Port_Data.Data_Transfer[3],0,S15C.Write.Port_1_Discrete_2_Reset_Count,0,8)BTD(Port_Data.Data_Transfer[4],0,S15C.Write.Port_1_Discrete_1_Reset_Count,24,8)BTD(Port_Data.Data_Transfer[5],0,S15C.Write.Port_1_Discrete_1_Reset_Count,16,8)BTD(Port_Data.Data_Transfer[6],0,S15C.Write.Port_1_Discrete_1_Reset_Count,8,8)BTD(Port_Data.Data_Transfer[7],0,S15C.Write.Port_1_Discrete_1_Reset_Count,0,8)BTD(Port_Data.Data_Transfer[9],1,S15C.Write.Port_1_Discrete_2,0,1)BTD(Port_Data.Data_Transfer[9],0,S15C.Write.Port_1_Discrete_1,0,1)OTU(Port_Data.Port_Read.[Port])OTL(Local_Control.6);
   42: NOP();
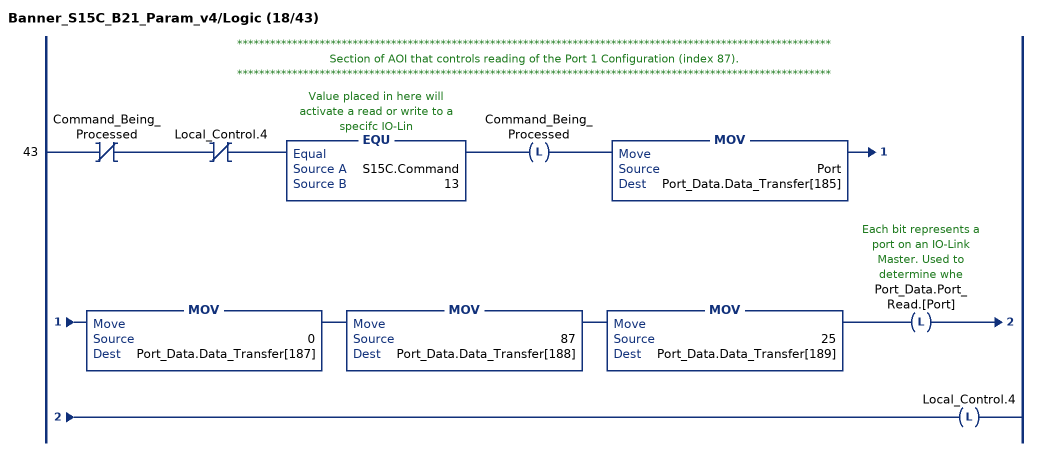
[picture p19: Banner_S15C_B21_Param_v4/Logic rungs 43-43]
   // ************************************************************************************************************
   // Section of AOI that controls reading of the Port 1 Configuration (index 87).
   // ************************************************************************************************************
   43: XIO(Command_Being_Processed)XIO(Local_Control.4)EQU(S15C.Command,13)OTL(Command_Being_Processed)MOV(Port,Port_Data.Data_Transfer[185])MOV(0,Port_Data.Data_Transfer[187])MOV(87,Port_Data.Data_Transfer[188])MOV(25,Port_Data.Data_Transfer[189])OTL(Port_Data.Port_Read.[Port])OTL(Local_Control.4);
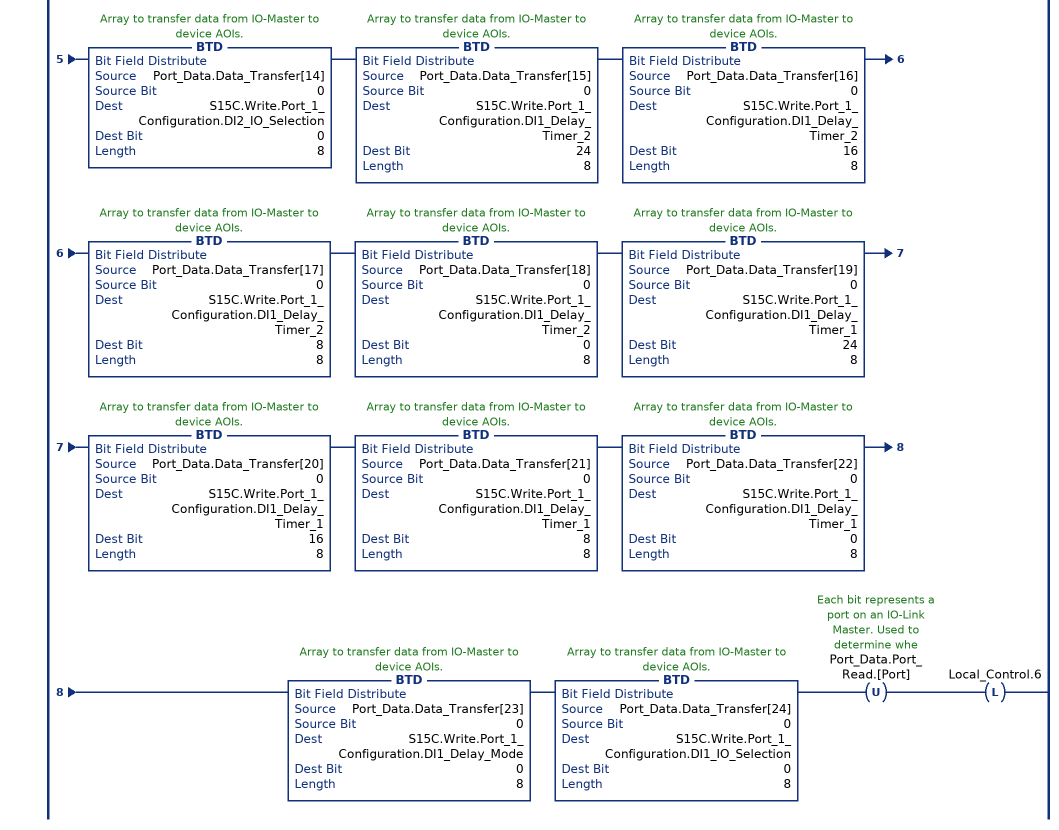
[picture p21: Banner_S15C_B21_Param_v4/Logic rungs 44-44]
   44: XIC(Local_Control.5)XIO(Local_Control.6)EQU(S15C.Command,13)BTD(Port_Data.Data_Transfer[0],0,S15C.Write.Port_1_Configuration.Counts_per_Minute_Mode,0,8)BTD(Port_Data.Data_Transfer[1],0,S15C.Write.Port_1_Configuration.Mirroring_Inversion,0,8)BTD(Port_Data.Data_Transfer[2],0,S15C.Write.Port_1_Configuration.Mirroring_Channel_Selection,0,8)BTD(Port_Data.Data_Transfer[3],0,S15C.Write.Port_1_Configuration.Mirroring_Port_Selection,0,8)BTD(Port_Data.Data_Transfer[4],0,S15C.Write.Port_1_Configuration.Mirroring_Enable,0,8)BTD(Port_Data.Data_Transfer[5],0,S15C.Write.Port_1_Configuration.DI2_Delay_Timer_2,24,8)BTD(Port_Data.Data_Transfer[6],0,S15C.Write.Port_1_Configuration.DI2_Delay_Timer_2,16,8)BTD(Port_Data.Data_Transfer[7],0,S15C.Write.Port_1_Configuration.DI2_Delay_Timer_2,8,8)BTD(Port_Data.Data_Transfer[8],0,S15C.Write.Port_1_Configuration.DI2_Delay_Timer_2,0,8)BTD(Port_Data.Data_Transfer[9],0,S15C.Write.Port_1_Configuration.DI2_Delay_Timer_1,24,8)BTD(Port_Data.Data_Transfer[10],0,S15C.Write.Port_1_Configuration.DI2_Delay_Timer_1,16,8)BTD(Port_Data.Data_Transfer[11],0,S15C.Write.Port_1_Configuration.DI2_Delay_Timer_1,8,8)BTD(Port_Data.Data_Transfer[12],0,S15C.Write.Port_1_Configuration.DI2_Delay_Timer_1,0,8)BTD(Port_Data.Data_Transfer[13],0,S15C.Write.Port_1_Configuration.DI2_Delay_Mode,0,8)BTD(Port_Data.Data_Transfer[14],0,S15C.Write.Port_1_Configuration.DI2_IO_Selection,0,8)BTD(Port_Data.Data_Transfer[15],0,S15C.Write.Port_1_Configuration.DI1_Delay_Timer_2,24,8)BTD(Port_Data.Data_Transfer[16],0,S15C.Write.Port_1_Configuration.DI1_Delay_Timer_2,16,8)BTD(Port_Data.Data_Transfer[17],0,S15C.Write.Port_1_Configuration.DI1_Delay_Timer_2,8,8)BTD(Port_Data.Data_Transfer[18],0,S15C.Write.Port_1_Configuration.DI1_Delay_Timer_2,0,8)BTD(Port_Data.Data_Transfer[19],0,S15C.Write.Port_1_Configuration.DI1_Delay_Timer_1,24,8)BTD(Port_Data.Data_Transfer[20],0,S15C.Write.Port_1_Configuration.DI1_Delay_Timer_1,16,8)BTD(Port_Data.Data_Transfer[21],0,S15C.Write.Port_1_Configuration.DI1_Delay_Timer_1,8,8)BTD(Port_Data.Data_Transfer[22],0,S15C.Write.Port_1_Configuration.DI1_Delay_Timer_1,0,8)BTD(Port_Data.Data_Transfer[23],0,S15C.Write.Port_1_Configuration.DI1_Delay_Mode,0,8)BTD(Port_Data.Data_Transfer[24],0,S15C.Write.Port_1_Configuration.DI1_IO_Selection,0,8)OTU(Port_Data.Port_Read.[Port])OTL(Local_Control.6);
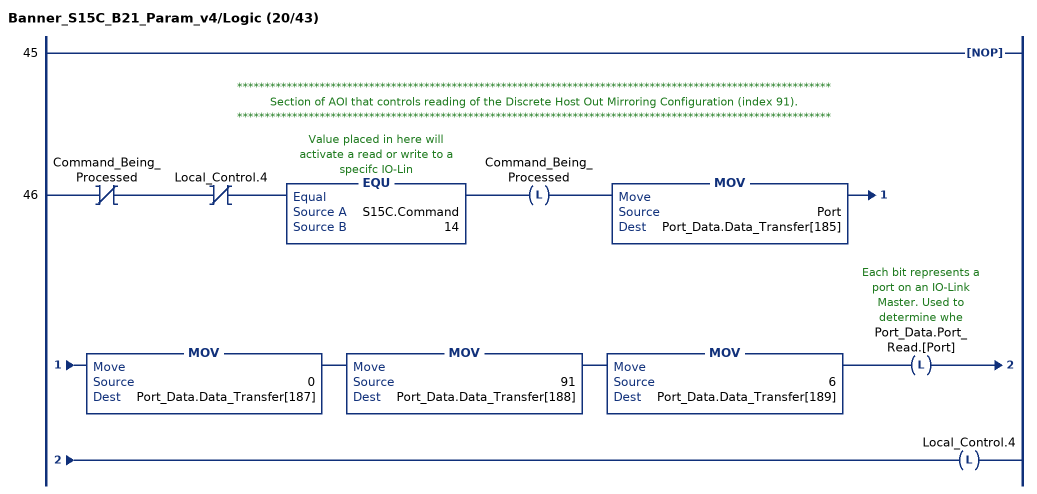
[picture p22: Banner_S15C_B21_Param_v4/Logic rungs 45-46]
   45: NOP();
   // ************************************************************************************************************
   // Section of AOI that controls reading of the Discrete Host Out Mirroring Configuration (index 91).
   // ************************************************************************************************************
   46: XIO(Command_Being_Processed)XIO(Local_Control.4)EQU(S15C.Command,14)OTL(Command_Being_Processed)MOV(Port,Port_Data.Data_Transfer[185])MOV(0,Port_Data.Data_Transfer[187])MOV(91,Port_Data.Data_Transfer[188])MOV(6,Port_Data.Data_Transfer[189])OTL(Port_Data.Port_Read.[Port])OTL(Local_Control.4);
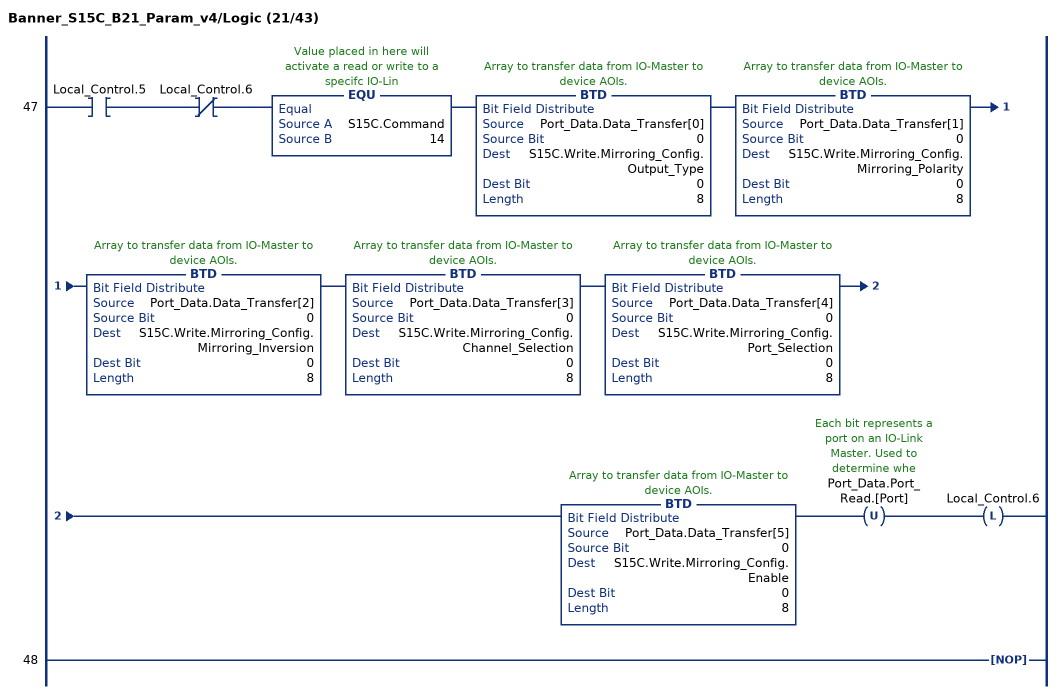
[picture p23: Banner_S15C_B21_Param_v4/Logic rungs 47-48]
   47: XIC(Local_Control.5)XIO(Local_Control.6)EQU(S15C.Command,14)BTD(Port_Data.Data_Transfer[0],0,S15C.Write.Mirroring_Config.Output_Type,0,8)BTD(Port_Data.Data_Transfer[1],0,S15C.Write.Mirroring_Config.Mirroring_Polarity,0,8)BTD(Port_Data.Data_Transfer[2],0,S15C.Write.Mirroring_Config.Mirroring_Inversion,0,8)BTD(Port_Data.Data_Transfer[3],0,S15C.Write.Mirroring_Config.Channel_Selection,0,8)BTD(Port_Data.Data_Transfer[4],0,S15C.Write.Mirroring_Config.Port_Selection,0,8)BTD(Port_Data.Data_Transfer[5],0,S15C.Write.Mirroring_Config.Enable,0,8)OTU(Port_Data.Port_Read.[Port])OTL(Local_Control.6);
   48: NOP();
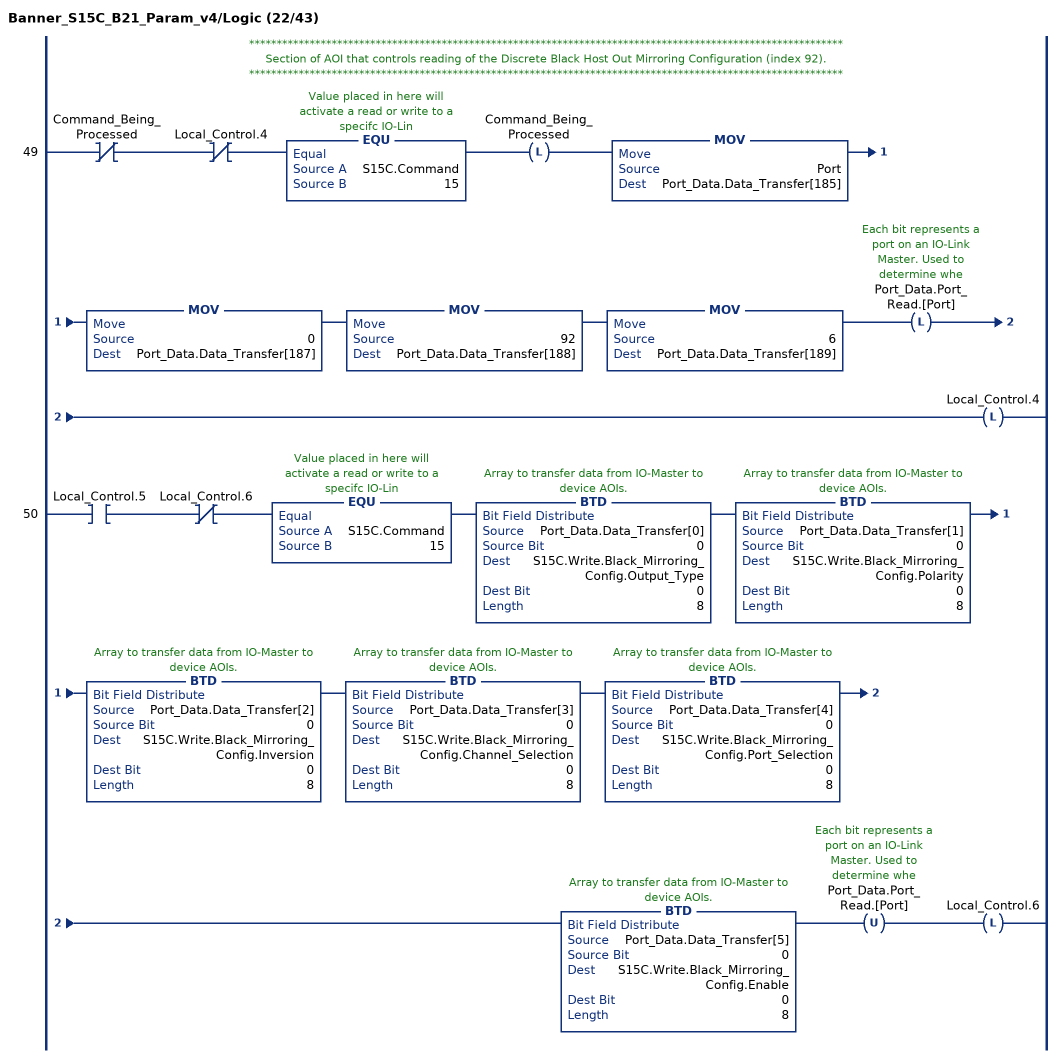
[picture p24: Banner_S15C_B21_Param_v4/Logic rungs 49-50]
   // ************************************************************************************************************
   // Section of AOI that controls reading of the Discrete Black Host Out Mirroring Configuration (index 92).
   // ************************************************************************************************************
   49: XIO(Command_Being_Processed)XIO(Local_Control.4)EQU(S15C.Command,15)OTL(Command_Being_Processed)MOV(Port,Port_Data.Data_Transfer[185])MOV(0,Port_Data.Data_Transfer[187])MOV(92,Port_Data.Data_Transfer[188])MOV(6,Port_Data.Data_Transfer[189])OTL(Port_Data.Port_Read.[Port])OTL(Local_Control.4);
   50: XIC(Local_Control.5)XIO(Local_Control.6)EQU(S15C.Command,15)BTD(Port_Data.Data_Transfer[0],0,S15C.Write.Black_Mirroring_Config.Output_Type,0,8)BTD(Port_Data.Data_Transfer[1],0,S15C.Write.Black_Mirroring_Config.Polarity,0,8)BTD(Port_Data.Data_Transfer[2],0,S15C.Write.Black_Mirroring_Config.Inversion,0,8)BTD(Port_Data.Data_Transfer[3],0,S15C.Write.Black_Mirroring_Config.Channel_Selection,0,8)BTD(Port_Data.Data_Transfer[4],0,S15C.Write.Black_Mirroring_Config.Port_Selection,0,8)BTD(Port_Data.Data_Transfer[5],0,S15C.Write.Black_Mirroring_Config.Enable,0,8)OTU(Port_Data.Port_Read.[Port])OTL(Local_Control.6);
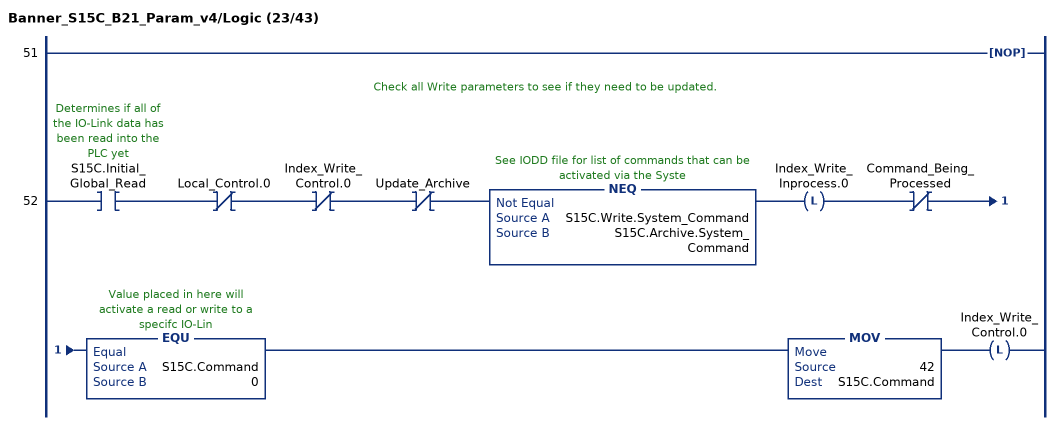
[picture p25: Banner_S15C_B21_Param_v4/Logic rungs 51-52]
   51: NOP();
   // Check all Write parameters to see if they need to be updated.
   52: XIC(S15C.Initial_Global_Read)XIO(Local_Control.0)XIO(Index_Write_Control.0)XIO(Update_Archive)NEQ(S15C.Write.System_Command,S15C.Archive.System_Command)OTL(Index_Write_Inprocess.0)XIO(Command_Being_Processed)EQU(S15C.Command,0)MOV(42,S15C.Command)OTL(Index_Write_Control.0);
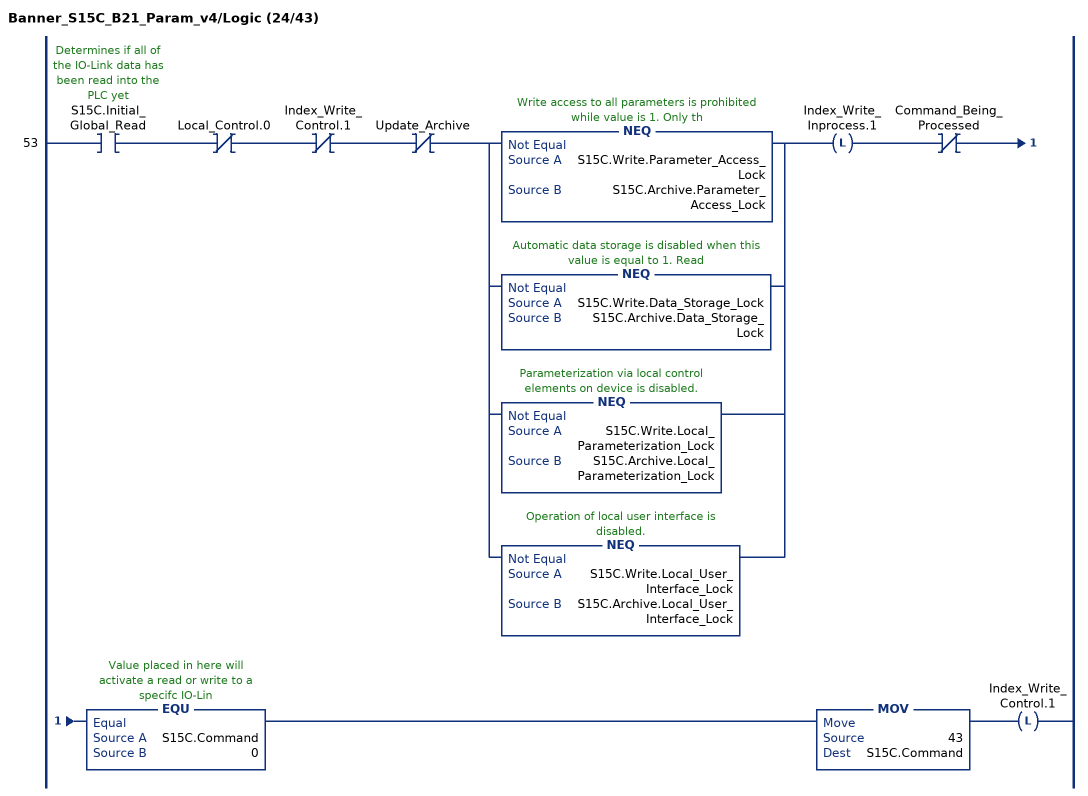
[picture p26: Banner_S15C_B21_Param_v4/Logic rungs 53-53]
   53: XIC(S15C.Initial_Global_Read)XIO(Local_Control.0)XIO(Index_Write_Control.1)XIO(Update_Archive)[NEQ(S15C.Write.Parameter_Access_Lock,S15C.Archive.Parameter_Access_Lock) ,NEQ(S15C.Write.Data_Storage_Lock,S15C.Archive.Data_Storage_Lock) ,NEQ(S15C.Write.Local_Parameterization_Lock,S15C.Archive.Local_Parameterization_Lock) ,NEQ(S15C.Write.Local_User_Interface_Lock,S15C.Archive.Local_User_Interface_Lock) ]OTL(Index_Write_Inprocess.1)XIO(Command_Being_Processed)EQU(S15C.Command,0)MOV(43,S15C.Command)OTL(Index_Write_Control.1);
